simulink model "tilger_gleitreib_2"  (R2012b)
settings: Solver=ode45  StartTime=0.0  StopTime=10.0  FixedStep=dt  MaxStep=dt  RelTol=1e-3
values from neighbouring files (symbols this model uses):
  c = 2200    [coulomb_1.m]    (also in coulomb_10.m = 0.1; coulomb_11.m = 0; coulomb_2.m; coulomb_3.m)
  FG = 500    [coulomb_1.m]    (also in coulomb_10.m = 10; coulomb_11.m = 10; coulomb_2.m; coulomb_3.m)
  FH = 12    [coulomb_10.m]    (also in coulomb_11.m; coulomb_3.m = 600; coulomb_4.m = 600; position_reg_1.m = 3.956)
  k = 10    [coulomb_10.m]    (also in coulomb_11.m; diff_filter_1.m = 250; diff_filter_2.m = 250; dry_friction_1.m = 2200)
  kT = k*mT/m,    [tilger_gleitreib2.m]    (also in unwucht_2.m = 5,; unwucht_3.m = 5,; unwucht_4.m = 5,; unwucht_5.m = 5,)
  m = 400    [coulomb_1.m]    (also in coulomb_10.m = 10; coulomb_11.m = 10; coulomb_2.m; coulomb_3.m)
  mT = 0.2*m    (= 20)    [tilger_gleitreib2.m]    (also in unwucht_2.m = 0.9*kT/(omega)^2,; unwucht_3.m = kT/(omega)^2,; unwucht_4.m = kT/(omegar)^2,; unwucht_5.m = kT/(omegar)^2,)
  sigma_0 = 5000    [position_reg_1.m]    (also in position_reg_2.m; slip_stick_21.m = 10000; slip_stick_s_12.m = 10000; tilger_gleitreib2.m = 1000)
  sigma_1 = sqrt(sigma_0)    [position_reg_1.m]    (also in position_reg_2.m; slip_stick_21.m = sqrt(1e5); slip_stick_s_12.m = sqrt(1e5); tilger_gleitreib2.m)
  sigma_2 = 0    [position_reg_1.m]    (also in position_reg_2.m; slip_stick_21.m; slip_stick_s_12.m; tilger_gleitreib2.m)
  v0 = 0    [coulomb_1.m]    (also in coulomb_2.m; coulomb_3.m; coulomb_4.m; coulomb_5.m)
  vs = 0.05    [position_reg_1.m]    (also in position_reg_2.m; slip_stick_21.m; slip_stick_3.m = 0.01; slip_stick_31.m)
  x0 = [1;0]*1e-2    [rad_aufhaeng_1.m]    (also in slip_stick_3_1.m = 0.1; slip_stick_3_11.m = 0.1; suspension_1.m = [1 1 1 1]'; tilger_gleitreib1.m = 0.2)

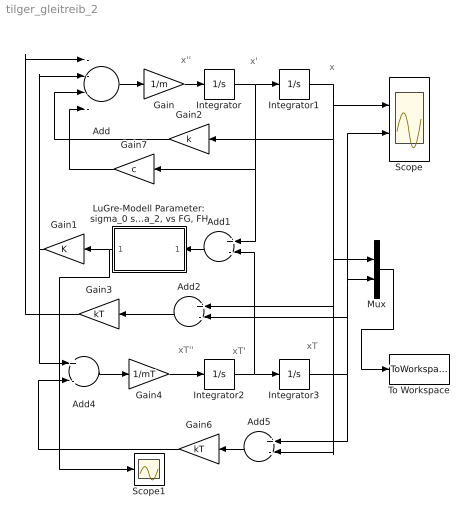
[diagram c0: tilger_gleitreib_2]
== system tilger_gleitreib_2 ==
  note: xT
  note: x
  note: x'
  note: x''
  note: xT'
  note: xT''
  Add : Sum  Inputs=----
  Add{1..2,4..5} (4 alike) : Sum  Inputs=+-
  Gain : Gain  Gain=1/m
  Gain1 : Gain
  Gain2 : Gain  Gain=k
  Gain3 : Gain  Gain=kT
  Gain4 : Gain  Gain=1/mT
  Gain6 : Gain  Gain=kT
  Gain7 : Gain  Gain=c
  Integrator : Integrator  InitialCondition=v0
  Integrator1 : Integrator  InitialCondition=x0
  Integrator2 : Integrator
  Integrator3 : Integrator
  "LuGre-Modell Parameter: sigma_0 sigma_1, sigma_2, vs FG, FH" : Subsystem
  Mux : Mux  Inputs=2
  Scope : Scope  NumInputPorts=2
  Scope1 : Scope
  To Workspace : ToWorkspace  VariableName=y  SampleTime=-1  SaveFormat=Structure With Time
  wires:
  Gain3/1 -> Add/1
  Add/1 -> Gain/1
  Integrator/1 -> Add1/1, Gain7/1, Integrator1/1
  Gain/1 -> Integrator/1
  Gain1/1 -> Add/2, Add4/1
  Gain2/1 -> Add/3
  Add2/1 -> Gain3/1
  Gain4/1 -> Integrator2/1
  Integrator2/1 -> Add1/2, Integrator3/1
  Integrator3/1 -> Scope/2, Mux/2, Add2/2, Add5/1
  Add4/1 -> Gain4/1
  Integrator1/1 -> Add5/2, Add2/1, Mux/1, Gain2/1, Scope/1
  Add5/1 -> Gain6/1
  Gain6/1 -> Add4/2
  Mux/1 -> To Workspace/1
  Add1/1 -> "LuGre-Modell Parameter: sigma_0 sigma_1, sigma_2, vs FG, FH"/1(v)
  Gain7/1 -> Add/4
  "LuGre-Modell Parameter: sigma_0 sigma_1, sigma_2, vs FG, FH"/1(Fr) -> Scope1/1, Gain1/1

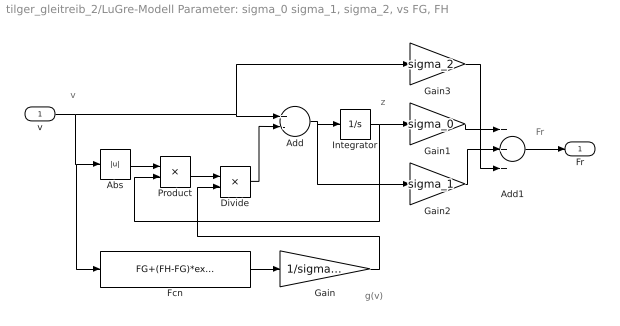
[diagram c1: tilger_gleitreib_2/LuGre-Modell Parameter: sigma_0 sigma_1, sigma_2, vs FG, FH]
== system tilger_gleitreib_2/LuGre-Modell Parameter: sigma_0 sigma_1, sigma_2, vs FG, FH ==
  note: z
  note: g(v)
  note: v
  note: Fr
  v : Inport
  Abs : Abs
  Add : Sum  Inputs=+-
  Add1 : Sum  Inputs=+++
  Divide : Product  Inputs=*/
  Fcn : Fcn  Expr=FG+(FH-FG)*exp(-(u/vs)^2)
  Gain : Gain  Gain=1/sigma_0
  Gain1 : Gain  Gain=sigma_0
  Gain2 : Gain  Gain=sigma_1
  Gain3 : Gain  Gain=sigma_2
  Integrator : Integrator
  Product : Product
  Fr : Outport
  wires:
  Product/1 -> Divide/1
  Gain/1 -> Divide/2
  Fcn/1 -> Gain/1
  Gain3/1 -> Add1/3
  Add1/1 -> Fr/1
  Gain1/1 -> Add1/1
  Divide/1 -> Add/2
  Abs/1 -> Product/1
  Gain2/1 -> Add1/2
  Add/1 -> Integrator/1, Gain2/1
  Integrator/1 -> Product/2, Gain1/1
  v/1 -> Abs/1, Fcn/1, Add/1, Gain3/1
